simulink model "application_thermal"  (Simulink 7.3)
settings: Solver=ode14x  StartTime=0.0  StopTime=6e3  RelTol=1e-3
StopFcn:
  | load temperatures.mat
  | plot(x(1,:), x(2,:),x(1,:), x(3,:),x(1,:), x(4,:),'*')
  | grid
  | axis([0 6000 -5 120])
  | title('Tranferts convectif, conductif et masse thermique')
  | xlabel('temps')
  | gtext('échelon d''entrée température')
  | gtext('température dans la matérieau')
libraries: fl_lib x8, nesl_utility x4

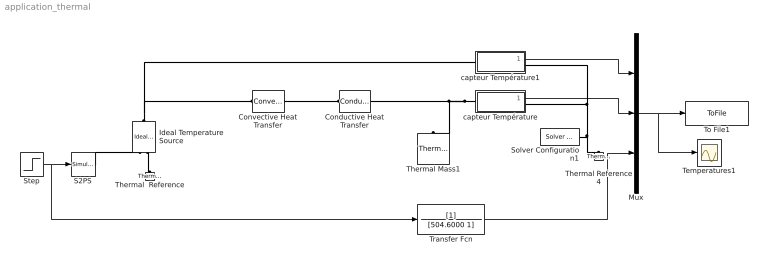
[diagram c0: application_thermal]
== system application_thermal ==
  Conductive Heat Transfer : fl_lib/Thermal/Thermal Elements/Conductive Heat Transfer  DialogController=NetworkEngine.DynNeDlgSource  SystemSampleTime=-1  area=5 m^2  thickness=0.1 m  th_cond=0.02 W/(m*K)  Q_Log=off  T_Log=off  LocalVarNames=|heat_flow|temperature_diff  LocalVarDescs=|Heat flow (J/s)|Temperature difference (K)  LocalVarLogging=[0 0]
  Convective Heat Transfer : fl_lib/Thermal/Thermal Elements/Convective Heat Transfer  DialogController=NetworkEngine.DynNeDlgSource  SystemSampleTime=-1  area=5 m^2  heat_tr_coeff=10 W/(m^2 * K)  Q_Log=off  T_Log=off  LocalVarNames=|heat_flow|temperature_diff  LocalVarDescs=|Heat flow (J/s)|Temperature difference (K)  LocalVarLogging=[0 0]
  Ideal Temperature Source : fl_lib/Thermal/Thermal Sources/Ideal Temperature Source  DialogController=NetworkEngine.DynNeDlgSource  SystemSampleTime=-1  Q_Log=off  T_Log=off  LocalVarNames=|Q|T  LocalVarDescs=|Q|T  LocalVarLogging=[0 0]
  Mux : Mux  Inputs=3
  S2PS : nesl_utility/Simulink-PS Converter  DialogController=NetworkEngine.DynNeUtilDlgSource  SystemSampleTime=-1  PhysicalDomain=network_engine_domain  LeftPortType=input  RightPortType=output  SubClassName=ps_input  Unit=1  AffineConversion=off  InputFilterTimeConstant=.001  UdotUserProvided=0
  Solver Configuration1 : nesl_utility/Solver Configuration  DialogController=NetworkEngine.DynNeUtilDlgSource  SystemSampleTime=-1  PhysicalDomain=network_engine_domain  LeftPortType=input  RightPortType=generic  SubClassName=solver  Accelerate=off  Profile=off  ResidualTolerance=1e-9  MaxNonlinIter=12  MaxModeIter=2  DoFixedCost=off  DoDC=off  LinearAlgebra=Sparse
  Step : Step  Time=3000  After=100  SampleTime=0
  Temperatures1 : Scope
  Thermal  Reference : fl_lib/Thermal/Thermal Elements/Thermal Reference  DialogController=NetworkEngine.DynNeDlgSource  SystemSampleTime=-1  Q_Log=off  LocalVarNames=|Q  LocalVarDescs=|Q  LocalVarLogging=[]
  Thermal Mass1 : fl_lib/Thermal/Thermal Elements/Thermal Mass  DialogController=NetworkEngine.DynNeDlgSource  SystemSampleTime=-1  mass=5 kg  sp_heat=100 J/kg/K  init_temp=0 C  Q_Log=off  LocalVarNames=|heat_flow|temperature  LocalVarDescs=|Heat flow (J/s)|Mass temperature (K)  LocalVarLogging=[0 0]
  Thermal Reference4 : fl_lib/Thermal/Thermal Elements/Thermal Reference  DialogController=NetworkEngine.DynNeDlgSource  SystemSampleTime=-1  Q_Log=off  LocalVarNames=|Q  LocalVarDescs=|Q  LocalVarLogging=[]
  To File1 : ToFile  Filename=temperatures  MatrixName=x
  Transfer Fcn : TransferFcn  Denominator=[504.6000 1]
  capteur Température : Subsystem
  capteur Température1 : Subsystem
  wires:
  Step/1 -> S2PS/1, Transfer Fcn/1
  capteur Température/1(T) -> Mux/2
  capteur Température1/1(T) -> Mux/1
  Mux/1 -> To File1/1, Temperatures1/1
  Transfer Fcn/1 -> Mux/3
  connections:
  Convective Heat Transfer/RConn1 -- Conductive Heat Transfer/LConn1
  S2PS/RConn1 -- Ideal Temperature Source/RConn1
  Ideal Temperature Source/RConn2 -- Thermal  Reference/LConn1
  capteur Température/LConn1 -- Conductive Heat Transfer/RConn1 -- Thermal Mass1/LConn1
  Ideal Temperature Source/LConn1 -- Convective Heat Transfer/LConn1 -- capteur Température1/LConn1
  capteur Température/RConn1 -- Thermal Reference4/LConn1 -- Solver Configuration1/RConn1 -- capteur Température1/RConn1

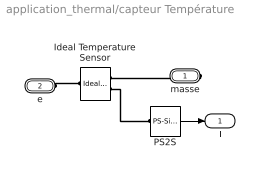
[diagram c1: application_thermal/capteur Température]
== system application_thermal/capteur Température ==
  Ideal Temperature Sensor : fl_lib/Thermal/Thermal Sensors/Ideal Temperature Sensor  DialogController=NetworkEngine.DynNeDlgSource  SystemSampleTime=-1  Qs_Log=off  Ts_Log=off  LocalVarNames=|Qs|Ts  LocalVarDescs=|Qs|Ts  LocalVarLogging=[0 0]
  PS2S : nesl_utility/PS-Simulink Converter  DialogController=NetworkEngine.DynNeUtilDlgSource  SystemSampleTime=-1  PhysicalDomain=network_engine_domain  LeftPortType=input  RightPortType=output  SubClassName=ps_output  Unit=1  AffineConversion=off
  masse : PMIOPort  Port=1  Side=Right
  e : PMIOPort  Port=2  Side=Left
  T : Outport
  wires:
  PS2S/1 -> T/1
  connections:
  e/RConn1 -- Ideal Temperature Sensor/LConn1
  masse/RConn1 -- Ideal Temperature Sensor/RConn1
  Ideal Temperature Sensor/RConn2 -- PS2S/LConn1

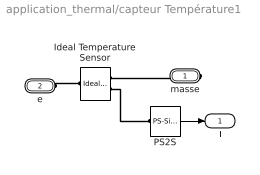
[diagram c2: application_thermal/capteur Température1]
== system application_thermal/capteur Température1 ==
  Ideal Temperature Sensor : fl_lib/Thermal/Thermal Sensors/Ideal Temperature Sensor  DialogController=NetworkEngine.DynNeDlgSource  SystemSampleTime=-1  Qs_Log=off  Ts_Log=off  LocalVarNames=|Qs|Ts  LocalVarDescs=|Qs|Ts  LocalVarLogging=[0 0]
  PS2S : nesl_utility/PS-Simulink Converter  DialogController=NetworkEngine.DynNeUtilDlgSource  SystemSampleTime=-1  PhysicalDomain=network_engine_domain  LeftPortType=input  RightPortType=output  SubClassName=ps_output  Unit=1  AffineConversion=off
  masse : PMIOPort  Port=1  Side=Right
  e : PMIOPort  Port=2  Side=Left
  T : Outport
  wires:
  PS2S/1 -> T/1
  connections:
  Ideal Temperature Sensor/RConn2 -- PS2S/LConn1
  masse/RConn1 -- Ideal Temperature Sensor/RConn1
  e/RConn1 -- Ideal Temperature Sensor/LConn1
